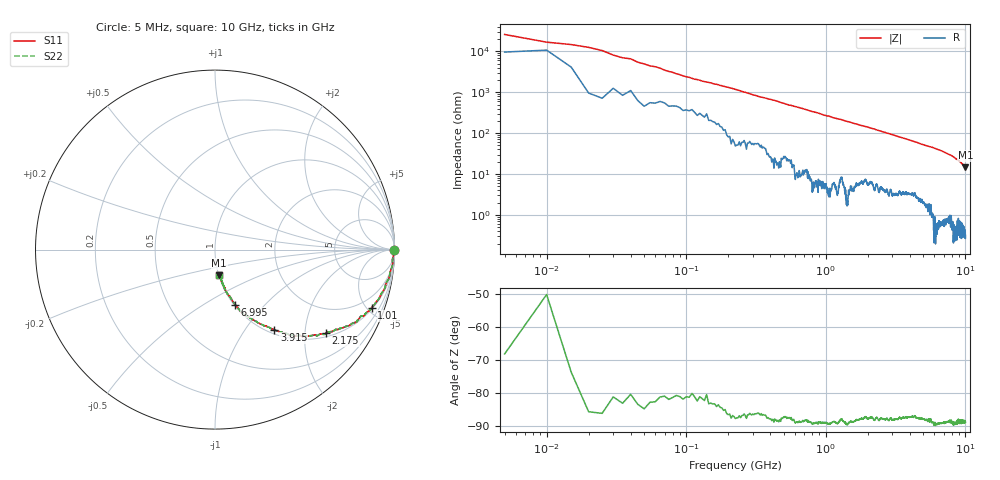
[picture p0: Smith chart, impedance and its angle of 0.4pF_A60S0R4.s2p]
! Amotech Co.,Ltd.
! http://www.amotech.co.kr/
! Part Number: A60S0R4
! These Parameters are Measured in Series Mode Connection
! Operation Temp=25[degC], DC Bias Voltage=0[V]
! Freq. Start=5[MHz] Stop=10[GHz], 2000[Steps]
! Date: Monday, July 13, 2020, 01:46:35
# GHZ S RI R 50.000000
!Freq.(Hz) S11(Real) S11(Imag) S21(Real) S21(Imag) S12(Real) S12(Imag) S22(Real) S22(Imag)
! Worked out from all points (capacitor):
!   2000 points, 5 MHz to 10 GHz, reference 50 ohm
!   read as one part in series: C = 665 fF near 55 MHz
!   lowest |Z| = 14.6 ohm at 10 GHz (marker M1)
!   S11 on the Smith chart (normalised r, x): 5 MHz: open; 1.01 GHz: 1.09, -5.35; 2.175 GHz: 1.11, -2.56; 3.915 GHz: 1.07, -1.38; 6.995 GHz: 1.01, -0.70; 10 GHz: 1.01, -0.29
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0.005  0.9985 -0.00359  0.00145 0.00359  0.00145 0.00359  0.9985 -0.00359
0.03  0.9979 -0.0122  0.00205 0.0122  0.00205 0.0122  0.9979 -0.0122
0.07  0.9947 -0.0282  0.00534 0.0282  0.00534 0.0282  0.9947 -0.0282
0.085  0.9931 -0.0345  0.00691 0.0345  0.00691 0.0345  0.9931 -0.0345
0.105  0.9916 -0.0422  0.00835 0.0422  0.00835 0.0422  0.9916 -0.0422
0.16  0.9887 -0.0619  0.0113 0.0619  0.0113 0.0619  0.9887 -0.0619
0.265  0.9847 -0.0977  0.0153 0.0977  0.0153 0.0977  0.9847 -0.0977
0.365  0.9739 -0.1328  0.0261 0.1328  0.0261 0.1328  0.9739 -0.1328
0.555  0.9505 -0.1959  0.0495 0.1959  0.0495 0.1959  0.9505 -0.1959
0.785  0.9174 -0.2645  0.0826 0.2645  0.0826 0.2645  0.9174 -0.2645
1.01  0.8736 -0.3244  0.1264 0.3244  0.1264 0.3244  0.8736 -0.3244
1.4  0.7902 -0.3994  0.2098 0.3994  0.2098 0.3994  0.7902 -0.3994
1.675  0.7259 -0.4299  0.2741 0.4299  0.2741 0.4299  0.7259 -0.4299
2.175  0.6174 -0.4654  0.3826 0.4654  0.3826 0.4654  0.6174 -0.4654
2.815  0.4926 -0.4845  0.5074 0.4845  0.5074 0.4845  0.4926 -0.4845
3.34  0.4035 -0.469  0.5965 0.469  0.5965 0.469  0.4035 -0.469
3.915  0.3313 -0.447  0.6687 0.447  0.6687 0.447  0.3313 -0.447
5.005  0.2222 -0.3964  0.7778 0.3964  0.7778 0.3964  0.2222 -0.3964
6.67  0.1271 -0.3249  0.8729 0.3249  0.8729 0.3249  0.1271 -0.3249
6.995  0.1131 -0.307  0.8869 0.307  0.8869 0.307  0.1131 -0.307
8.335  0.0633 -0.237  0.9367 0.237  0.9367 0.237  0.0633 -0.237
10  0.0239 -0.1422  0.9761 0.1422  0.9761 0.1422  0.0239 -0.1422
